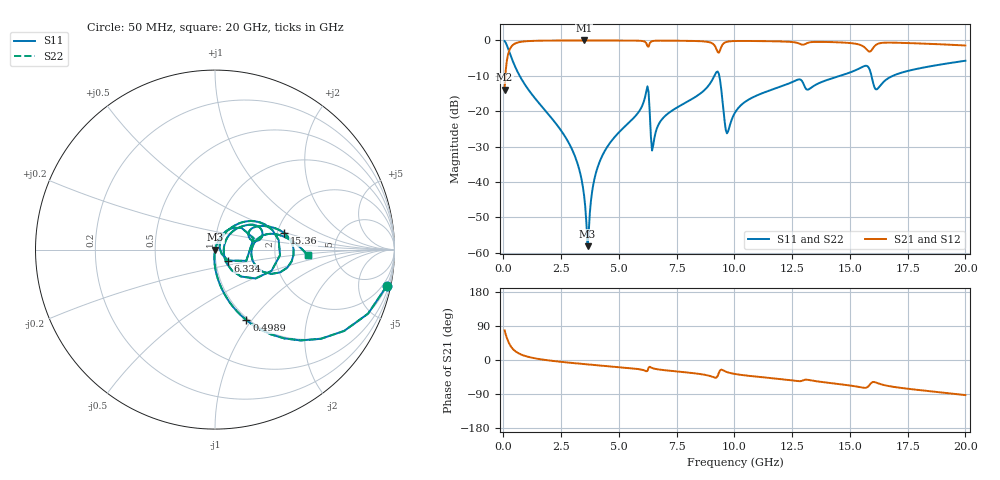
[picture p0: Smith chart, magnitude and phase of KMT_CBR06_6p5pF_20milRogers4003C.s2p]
! Data measured by Modelithics Inc. support@modelithics.com 813-866-6335
! KEMET CBR0603 6.5pF, Pad Width= 0.851mm, Pad Length= 0.64mm, Pad Gap= 0.62mm, 20mil Rogers 4003C substrate Data, January 2022
# hz S ma R 50
! 2 Port Network Data from SP1.SP block
! freq  magS11  angS11  magS21  angS21  magS12  angS12  magS22  angS22
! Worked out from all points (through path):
!   401 points, 50 MHz to 20 GHz, reference 50 ohm
!   highest |S21| = -0.01 dB at 3.491 GHz (marker M1); lowest = -13.9 dB at 50 MHz (marker M2)
!   group delay of S21, straight-line fit = 14.3 ps
!   lowest |S11| = -58.1 dB at 3.641 GHz (marker M3), VSWR 1.00, Z = 50.1 - j0.0625 ohm
!   |S11| at or under -10 dB: 702.1 MHz to 9.133 GHz (8.431 GHz wide, 171 % of centre); 9.343 GHz to 14.57 GHz (5.232 GHz wide, 43.8 % of centre); 15.93 GHz to 16.86 GHz (925.8 MHz wide, 5.65 % of centre)
!   |S22| runs from -58.1 to -0.2 dB; largest |S21 - S12| = 0
!   S11 on the Smith chart (normalised r, x): 50 MHz: 0.98, -9.57; 498.9 MHz: 0.98, -0.94; 6.334 GHz: 1.15, -0.14; 15.36 GHz: 2.17, +0.48; 20 GHz: 3.11, -0.26
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5e7  0.9794 -11.8  0.2019 78.2  0.2019 78.2  0.9794 -11.8
4.98875e8  0.4309 -66.0  0.9018 23.9  0.9018 23.9  0.4309 -66.0
2.74325e9  0.03992 -95.0  0.9981 -6.4  0.9981 -6.4  0.03992 -95.0
3.391625e9  0.01046 -94.0  0.9987 -10.2  0.9987 -10.2  0.01046 -94.0
3.491375e9  0.006437 -90.5  0.9987 -10.7  0.9987 -10.7  0.006437 -90.5
3.641e9  0.001242 -30.2  0.9987 -11.5  0.9987 -11.5  0.001242 -30.2
3.990125e9  0.01295 71.1  0.9985 -13.4  0.9985 -13.4  0.01295 71.1
4.389125e9  0.02755 71.7  0.9981 -15.5  0.9981 -15.5  0.02755 71.7
6.184625e9  0.1911 39.0  0.9148 -29.8  0.9148 -29.8  0.1911 39.0
6.33425e9  0.09477 -40.2  0.9114 -18.0  0.9114 -18.0  0.09477 -40.2
6.483875e9  0.03301 38.3  0.9831 -22.2  0.9831 -22.2  0.03301 38.3
6.73325e9  0.06659 60.2  0.9921 -25.1  0.9921 -25.1  0.06659 60.2
9.227e9  0.3587 8.7  0.7491 -46.1  0.7491 -46.1  0.3587 8.7
9.675875e9  0.0487 -2.9  0.9567 -31.8  0.9567 -31.8  0.0487 -2.9
1.0025e10  0.09549 44.2  0.9804 -36.9  0.9804 -36.9  0.09549 44.2
1.271825e10  0.2774 26.5  0.9234 -55.7  0.9234 -55.7  0.2774 26.5
1.336662e10  0.2198 28.7  0.9486 -54.3  0.9486 -54.3  0.2198 28.7
1.536162e10  0.3951 13.6  0.8812 -70.9  0.8812 -70.9  0.3951 13.6
1.591025e10  0.3397 -23.5  0.7093 -61.4  0.7093 -61.4  0.3397 -23.5
1.615962e10  0.2034 -1.3  0.879 -60.1  0.879 -60.1  0.2034 -1.3
1.670825e10  0.2986 16.5  0.9311 -69.1  0.9311 -69.1  0.2986 16.5
2e10  0.5164 -3.5  0.8477 -92.6  0.8477 -92.6  0.5164 -3.5
